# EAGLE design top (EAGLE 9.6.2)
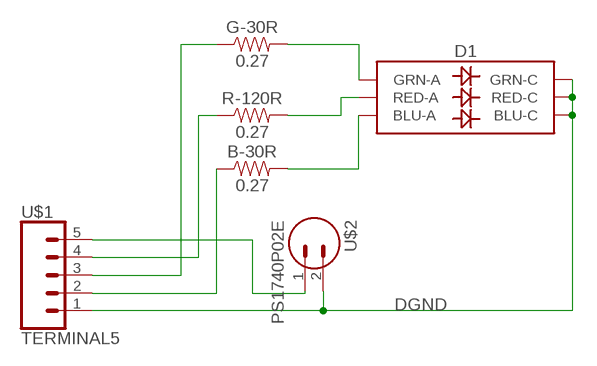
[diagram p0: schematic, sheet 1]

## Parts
B-30R  0.27  0.27OHM-0603-1/10W-1%  [0603]
D1  LED-RGBBRG  [LED-TRICOLOR-5050]
G-30R  0.27  0.27OHM-0603-1/10W-1%  [0603]
R-120R  0.27  0.27OHM-0603-1/10W-1%  [0603]
U$1  TERMINAL5  [1X5]
U$2  PS1740P02E  [PS1740]

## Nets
DGND: D1.1(BLU-C) D1.3(RED-C) D1.5(GRN-C) U$1.1 U$2.2
N$1: U$1.5 U$2.1
N$2: B-30R.1 U$1.2
N$3: R-120R.1 U$1.4
N$4: G-30R.1 U$1.3
N$5: B-30R.2 D1.2(BLU-A)
N$6: D1.4(RED-A) R-120R.2
N$7: D1.6(GRN-A) G-30R.2

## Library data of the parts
B-30R G-30R R-120R = SparkFun-Resistors:0.27OHM: 0.27Ω resistor; PROD_ID: RES-08787
D1 = habits:LED-RGB: LED-RGB 6 pin RGB LED (no common connector) Packages: PLCC-6 LED-TRICOLOR-5050 - No built-in IC SparkFun Products: Digital Sandbox LED- SMD RGB; PROD_ID: DIO-16048
U$1 = habits:TERMINAL5
U$2 = habits:PS1740P02E

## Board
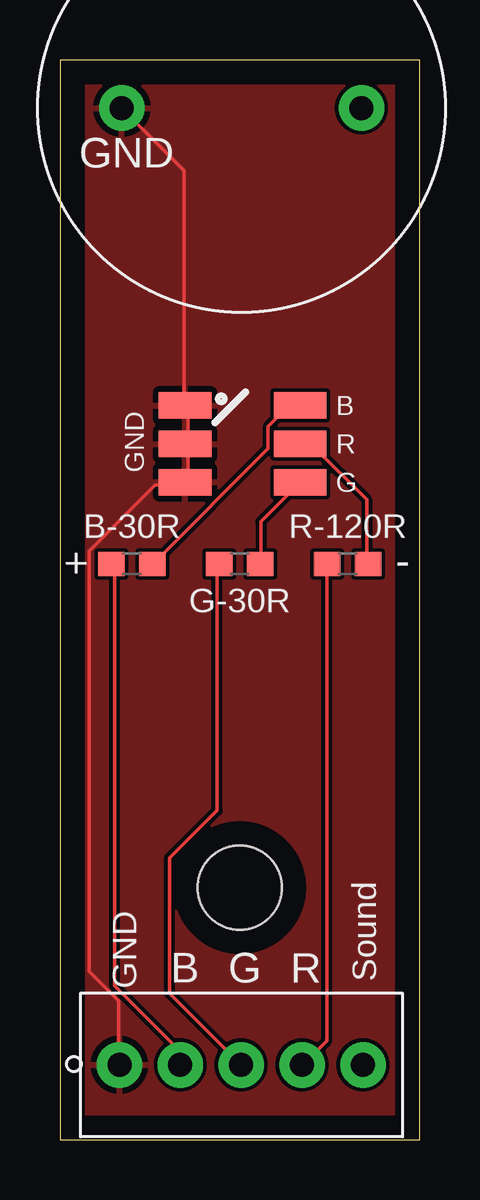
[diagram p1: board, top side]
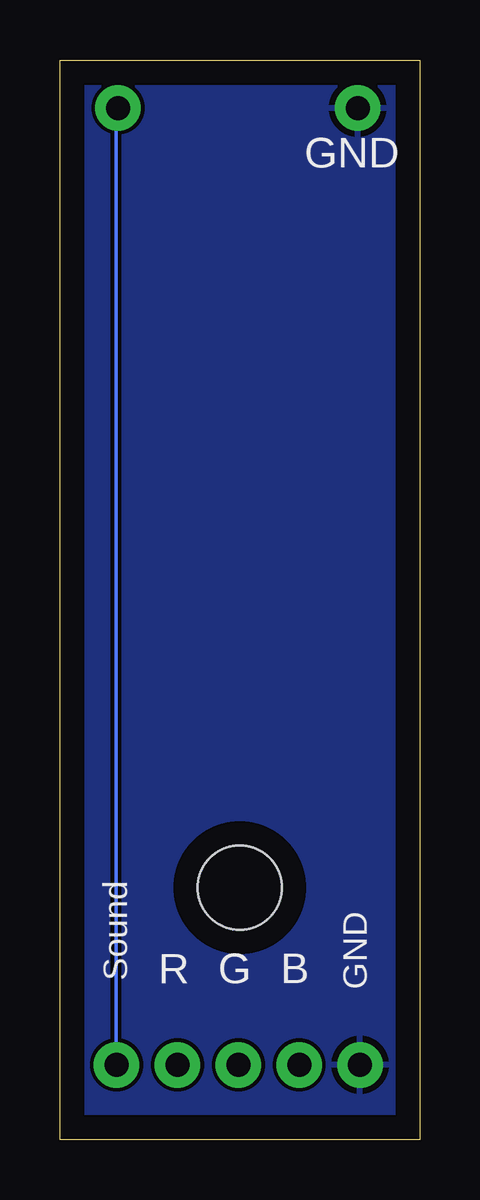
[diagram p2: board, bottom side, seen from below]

Size 15 x 45 mm. Coordinates in mm from the lower left corner, seen from the top.
Outline: 0,0 15,0 15,45 0,45 0,0
Copper layers (1*16): Top 0.035mm / dielectric 1.5mm / Bottom 0.035mm
Design rules "default": minimum track width 6mil, minimum drill 0.35mm, track to track 6mil, track to pad 6mil, pad to pad 6mil, via to via 6mil, smd to smd 6mil, copper to edge 40mil, drill to drill 6mil, minimum pad ring 10mil, minimum via ring 8mil, stop-mask expansion 4mil, vias tented up to drill 0mil, thermal gap 10mil
Holes 3.5 mm at 7.5,10.5

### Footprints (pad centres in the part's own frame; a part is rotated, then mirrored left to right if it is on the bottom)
0603 = smd 1.1 x 1: 1 -0.85,0; 2 0.85,0
LED-TRICOLOR-5050 = smd 2.2 x 1.1: 1 2.781,-1.6; 2 -2.019,-1.6; 3 2.781,0; 4 -2.019,0; 5 2.781,1.6; 6 -2.019,1.6
1X5 = drill 1 pad 1.9: 1 0,0; 2 2.54,0; 3 5.08,0; 4 7.62,0; 5 10.16,0
PS1740 = drill 1 pad 1.9: 1 0,0; 2 10,0

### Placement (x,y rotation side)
B-30R  3,24 0 top
D1  8,29 180 top
G-30R  7.5,24 0 top
R-120R  12,24 0 top
U$1  2.48,3.11 0 top
U$2  12.58,43 180 top

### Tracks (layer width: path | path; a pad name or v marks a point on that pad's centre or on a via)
DGND
  Top 0.152: U$2.2 2.59,42.98 5.18,40.39 5.18,30.63 D1.1 5.33,30.48 5.33,29.11 D1.3 5.33,28.96 5.33,27.43 D1.5 5.18,27.28 3.96,27.28 1.22,24.54 1.22,7.01 2.44,5.79 2.44,3.2 U$1.1
  pour Top: 0,0 15,0 15,45 0,45
  pour Bottom: 0,0 15,0 15,45 0,45
N$1
  Bottom 0.152: U$2.1 12.65,42.98 12.65,3.2 U$1.5
N$2
  Top 0.152: B-30R.1 2.29,23.93 2.29,6.4 4.88,3.81 4.88,3.2 U$1.2
N$3
  Top 0.152: R-120R.1 11.12,23.93 11.12,4.12 10.21,3.2 U$1.4
N$4
  Top 0.152: G-30R.1 6.55,23.93 6.55,13.72 4.57,11.73 4.57,6.1 7.47,3.2 U$1.3
N$5
  Top 0.152: B-30R.2 3.96,24.08 8.69,28.8 8.69,29.72 9.45,30.48 9.91,30.48 D1.2
N$6
  Top 0.152: R-120R.2 12.8,24.08 12.8,26.67 10.52,28.96 10.06,28.96 D1.4
N$7
  Top 0.152: G-30R.2 8.38,24.08 8.38,25.76 9.91,27.28 D1.6

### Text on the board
tPlace: GND | B | R | GND | G | - | + | B | G | R | Sound | GND
bPlace: GND | Sound | GND | B | G | R

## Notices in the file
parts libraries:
SparkFun-Resistors: Licensing: Creative Commons ShareAlike 4.0 International - https://creativecommons.org/licenses/by-sa/4.0
